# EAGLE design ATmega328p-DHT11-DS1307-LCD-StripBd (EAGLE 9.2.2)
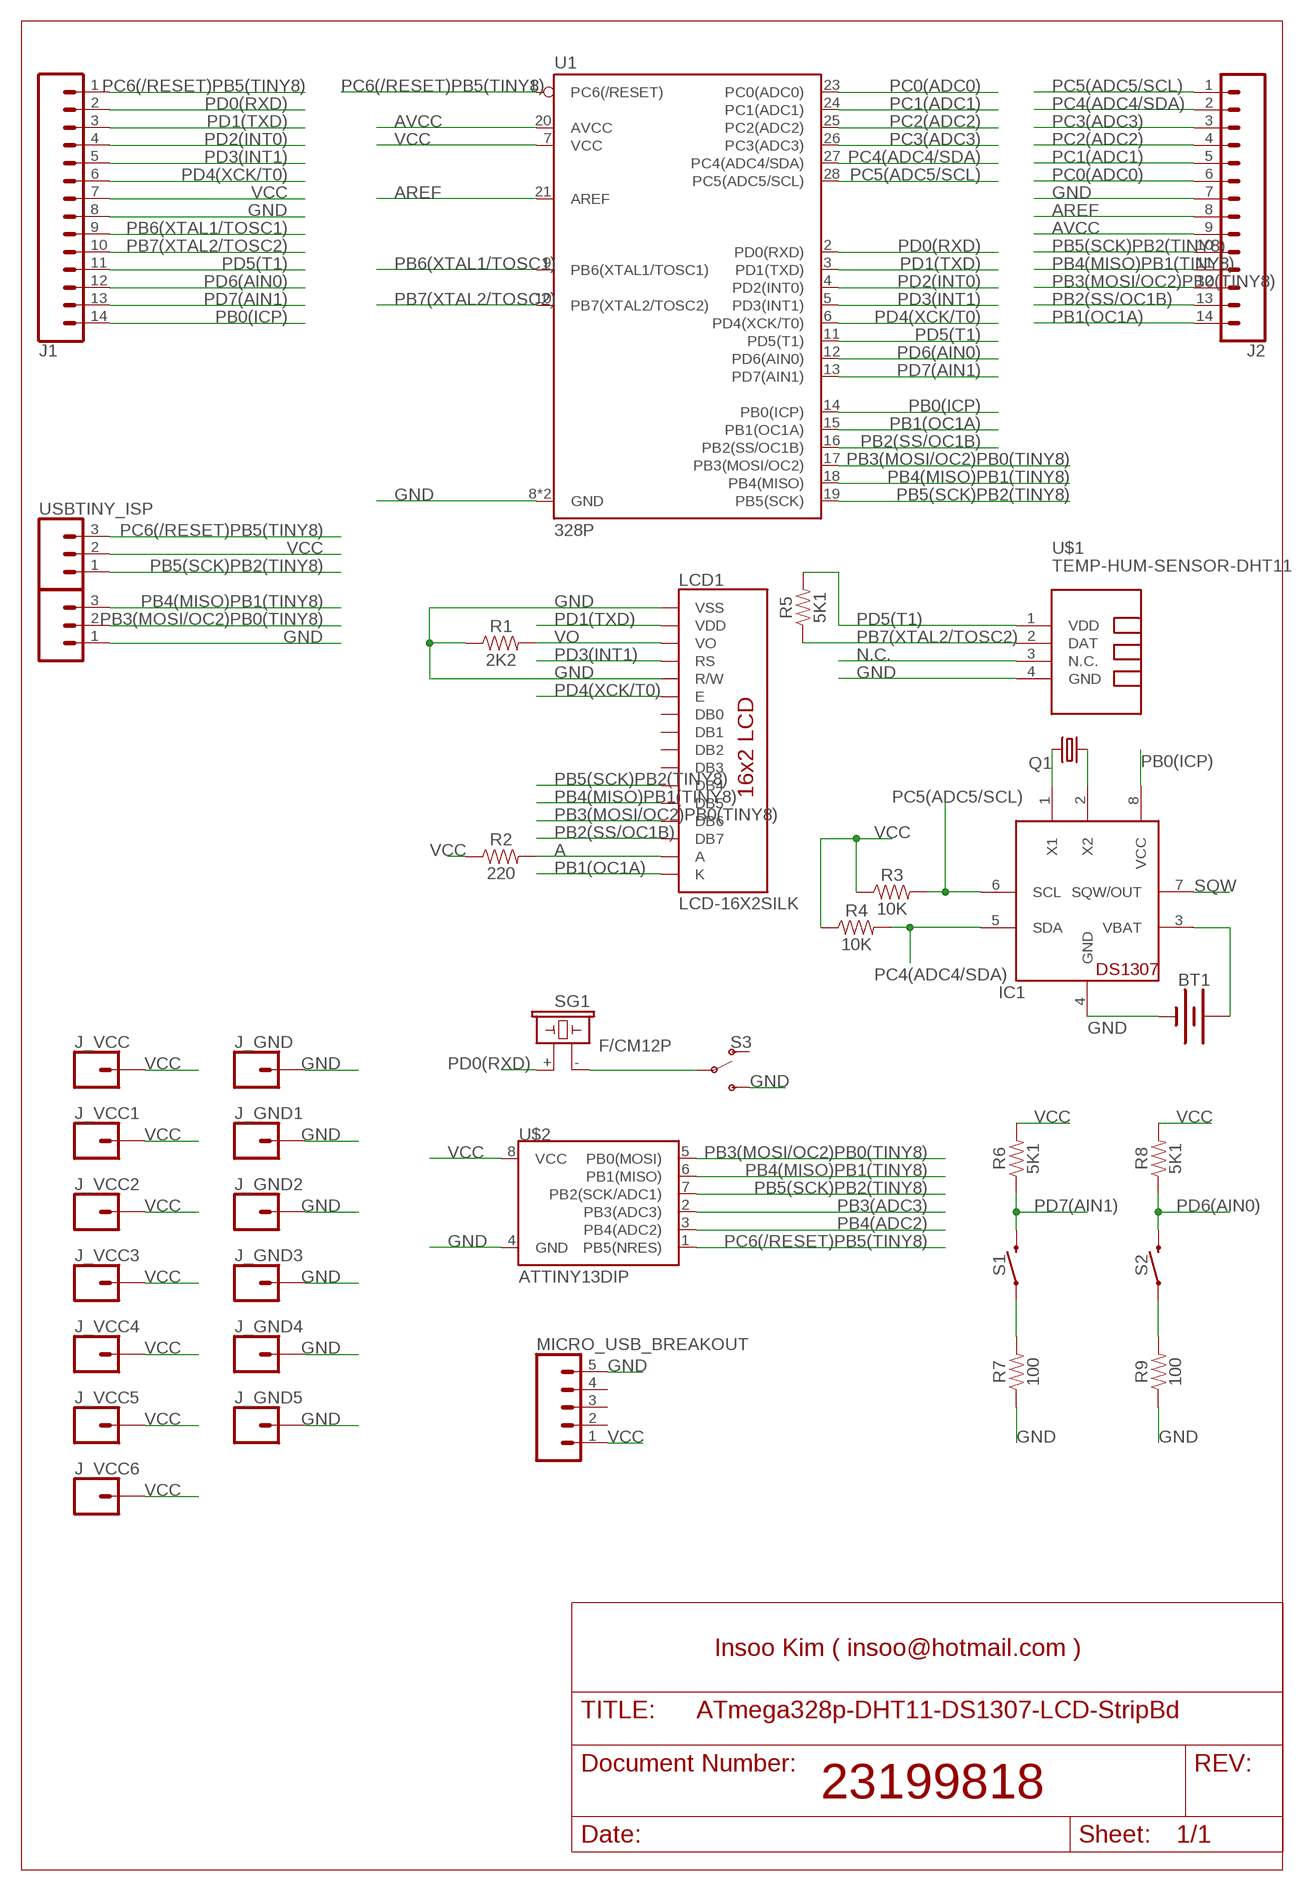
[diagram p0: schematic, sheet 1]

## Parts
BT1  BATTERY-20MM_PTH  [BATTCOM_20MM_PTH]
IC1  DS1307  [DIL08]
J1  CONN_14  [1X14]
J2  CONN_14  [1X14]
J3  455-1750-1-ND  CONN_03  [1X03]
J_GND  CONN_01  [1X01]
J_GND1  CONN_01  [1X01]
J_GND2  CONN_01  [1X01]
J_GND3  CONN_01  [1X01]
J_GND4  CONN_01  [1X01]
J_GND5  CONN_01  [1X01]
J_VCC  CONN_01  [1X01]
J_VCC1  CONN_01  [1X01]
J_VCC2  CONN_01  [1X01]
J_VCC3  CONN_01  [1X01]
J_VCC4  CONN_01  [1X01]
J_VCC5  CONN_01  [1X01]
J_VCC6  CONN_01  [1X01]
LCD1  LCD-16X2SILK  [LCD-16X2]
MICRO_USB_BREAKOUT  CONN_05  [1X05]
Q1  CRYSTALTC26H  [TC26H]
R1  2K2  1KOHM-HORIZ-1/4W-5%  [AXIAL-0.3]
R2  220  1KOHM-HORIZ-1/4W-5%  [AXIAL-0.3]
R3  10K  1KOHM-HORIZ-1/4W-5%  [AXIAL-0.3]
R4  10K  1KOHM-HORIZ-1/4W-5%  [AXIAL-0.3]
R5  5K1  1KOHM-HORIZ-1/4W-5%  [AXIAL-0.3]
R6  5K1  1KOHM-HORIZ-1/4W-5%  [AXIAL-0.3]
R7  100  1KOHM-HORIZ-1/4W-5%  [AXIAL-0.3]
R8  5K1  1KOHM-HORIZ-1/4W-5%  [AXIAL-0.3]
R9  100  1KOHM-HORIZ-1/4W-5%  [AXIAL-0.3]
S1  MOMENTARY-SWITCH-SPST-PTH-12MM  [TACTILE_SWITCH_PTH_12MM]
S2  MOMENTARY-SWITCH-SPST-PTH-12MM  [TACTILE_SWITCH_PTH_12MM]
S3  SWITCH-SPDT-PTH-11.6X4.0MM  [SWITCH_SPDT_PTH_11.6X4.0MM]
SG1  F/CM12P  [F/CM12P]
U1  328P  ATMEGA328P_PDIP  [DIP28]
U$1  TEMP-HUM-SENSOR-DHT11  [TEMP-HUM-SENSOR-DHT11]
U$2  ATTINY13DIP  [DIP08_MCU]
USBTINY_ISP  455-1750-1-ND  CONN_03  [1X03]

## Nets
A: LCD1.15(A) R2.P$2
AREF: J2.8 U1.21(AREF)
AVCC: J2.9 U1.20(AVCC)
GND: BT1.2(-) IC1.4(GND) J1.8 J2.7 J3.1 J_GND1.1 J_GND2.1 J_GND3.1 J_GND4.1 J_GND5.1 J_GND.1 LCD1.1(VSS) LCD1.5(R/W) MICRO_USB_BREAKOUT.5 R1.P$1 R7.P$1 R9.P$1 S3.3(S) U1.8(GND) U1.22(GND) U$1.4(GND) U$2.4(GND)
N$2: S3.2(P) SG1.-
N$40: R7.P$2 S1.1
N$54: IC1.2(X2) Q1.1
N$55: IC1.1(X1) Q1.2
N$56: R9.P$2 S2.1
N$58: BT1.1(+) IC1.3(VBAT)
N.C.: U$1.3(N.C.)
PB0(ICP): IC1.8(VCC) J1.14 U1.14(PB0(ICP))
PB1(OC1A): J2.14 LCD1.16(K) U1.15(PB1(OC1A))
PB2(SS/OC1B): J2.13 LCD1.14(DB7) U1.16(PB2(SS/OC1B))
PB3(ADC3): U$2.2(PB3(ADC3))
PB3(MOSI/OC2)PB0(TINY8): J2.12 J3.2 LCD1.13(DB6) U1.17(PB3(MOSI/OC2)) U$2.5(PB0(MOSI))
PB4(ADC2): U$2.3(PB4(ADC2))
PB4(MISO)PB1(TINY8): J2.11 J3.3 LCD1.12(DB5) U1.18(PB4(MISO)) U$2.6(PB1(MISO))
PB5(SCK)PB2(TINY8): J2.10 LCD1.11(DB4) U1.19(PB5(SCK)) U$2.7(PB2(SCK/ADC1)) USBTINY_ISP.1
PB6(XTAL1/TOSC1): J1.9 U1.9(PB6(XTAL1/TOSC1))
PB7(XTAL2/TOSC2): J1.10 R5.P$1 U1.10(PB7(XTAL2/TOSC2)) U$1.2(DAT)
PC0(ADC0): J2.6 U1.23(PC0(ADC0))
PC1(ADC1): J2.5 U1.24(PC1(ADC1))
PC2(ADC2): J2.4 U1.25(PC2(ADC2))
PC3(ADC3): J2.3 U1.26(PC3(ADC3))
PC4(ADC4/SDA): IC1.5(SDA) J2.2 R4.P$2 U1.27(PC4(ADC4/SDA))
PC5(ADC5/SCL): IC1.6(SCL) J2.1 R3.P$2 U1.28(PC5(ADC5/SCL))
PC6(/RESET)PB5(TINY8): J1.1 U1.1(PC6(/RESET)) U$2.1(PB5(NRES)) USBTINY_ISP.3
PD0(RXD): J1.2 SG1.+ U1.2(PD0(RXD))
PD1(TXD): J1.3 LCD1.2(VDD) U1.3(PD1(TXD))
PD2(INT0): J1.4 U1.4(PD2(INT0))
PD3(INT1): J1.5 LCD1.4(RS) U1.5(PD3(INT1))
PD4(XCK/T0): J1.6 LCD1.6(E) U1.6(PD4(XCK/T0))
PD5(T1): J1.11 R5.P$2 U1.11(PD5(T1)) U$1.1(VDD)
PD6(AIN0): J1.12 R8.P$1 S2.3 U1.12(PD6(AIN0))
PD7(AIN1): J1.13 R6.P$1 S1.3 U1.13(PD7(AIN1))
SQW: IC1.7(SQW/OUT)
VCC: J1.7 J_VCC1.1 J_VCC2.1 J_VCC3.1 J_VCC4.1 J_VCC5.1 J_VCC6.1 J_VCC.1 MICRO_USB_BREAKOUT.1 R2.P$1 R3.P$1 R4.P$1 R6.P$2 R8.P$2 U1.7(VCC) U$2.8(VCC) USBTINY_ISP.2
VO: LCD1.3(VO) R1.P$2
Unconnected: LCD1.7(DB0) LCD1.8(DB1) LCD1.9(DB2) LCD1.10(DB3) MICRO_USB_BREAKOUT.2 MICRO_USB_BREAKOUT.3 MICRO_USB_BREAKOUT.4 S3.1(O)

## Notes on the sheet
- Insoo Kim ( insoo@hotmail.com )
- 23199818

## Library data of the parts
BT1 = SparkFun-Batteries:BATTERY: Battery - Single Cell; PROD_ID: BATT-09031; SF_SKU: PRT-00783
IC1 = adafruit:DS1307: DS1307 Real time clock (RTC) with battery backup ability. Talk to it via i2c
J1 J2 = SparkFun-Connectors:CONN_14: Multi connection point. Often used as Generic Header-pin footprint for 0.1 inch spaced/style header connections On any of the 0.1 inch spaced packages, you can populate with these: Break Away Headers - Straight (PRT-00116) Break Away Male Headers - Right Angle (PRT-00553) Female Headers (PRT-00115)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
J3 USBTINY_ISP = SparkFun-Connectors:CONN_03: Multi connection point. Often used as Generic Header-pin footprint for 0.1 inch spaced/style header connections On any of the 0.1 inch spaced packages, you can populate with these: Break Away Headers - Straight (PRT-00116) Break Away Male Headers - Right Angle (PRT-00553) Female Headers (PRT-00115)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; PROD_ID: XXX-00000
J_GND J_GND1-J_GND5 J_VCC J_VCC1-J_VCC6 = SparkFun-Connectors:CONN_01: Single connection point. Often used as Generic Header-pin footprint for 0.1 inch spaced/style header connections
LCD1 = SparkFun-Displays:LCD-16X2: Standard text-only 16x2 parallel input LCD Basic 16 character by 2 line display. Typically utilizes the extremely common HD44780 parallel interface chipset SparkFun Products: Basic 16x2 Green Basic 8x2 Green; SF_ID: LCD-00255
MICRO_USB_BREAKOUT = SparkFun-Connectors:CONN_05: Multi connection point. Often used as Generic Header-pin footprint for 0.1 inch spaced/style header connections On any of the 0.1 inch spaced packages, you can populate with these: Break Away Headers - Straight (PRT-00116) Break Away Male Headers - Right Angle (PRT-00553) Female Headers (PRT-00115)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
Q1 = adafruit:CRYSTAL: CRYSTAL; OC_FARNELL: unknown; OC_NEWARK: unknown
R1-R9 = SparkFun-Resistors:1KOHM: 1kΩ resistor; PROD_ID: RES-08380; VALUE: 1k
S1 S2 = SparkFun-Switches:MOMENTARY-SWITCH-SPST: Momentary Switch (Pushbutton) - SPST; PROD_ID: SWCH-09185; SF_SKU: COM-09190
S3 = SparkFun-Switches:SWITCH-SPDT: Single Pole, Double Throw (SPDT) Switch Single-pole, double-throw (SPDT) switch. Variant Overview SMD-AYZ0202 Surface Mount DPDT Switch (COM-00597) Used on e.g. LilyPad Arduino USB - ATmega32U4 Board PTH-11.6X4.0MM SPDT Mini Power Switch (COM-00102) Used on e.g. SparkFun Simon Says - Through-Hole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; PROD_ID: SWCH-08261; SF_SKU: COM-00102
SG1 = buzzer:F/CM12P: BUZZER; OC_FARNELL: unknown; OC_NEWARK: unknown
U1 = SparkFun-IC-Microcontroller:ATMEGA328P_PDIP: Atmel 328P Through hole ATMEGA328P uC used in the Arduino 32kb flash, 1k EEPROM, 2k SRAM Datasheet SparkFun Products Storefront component: AVR 28 Pin 20MHz 32K 6A/D - ATMega328P (COM-09061) SparkFun Simon Says - Through-Hole Soldering Kit (KIT-10547) SparkFun Learn to Solder - Simon Says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; PROD_ID: IC-09136
U$1 = diy-modules:TEMP-HUM-SENSOR-DHT11: DHT11 - digital humidity & temperature sensor DHT11 datasheet available here: https://akizukidenshi.com/download/ds/aosong/DHT11.pdf Click here to find device on ebay.com
U$2 = SparkFun-Retired:ATTINY13: ATTINY13 Retired

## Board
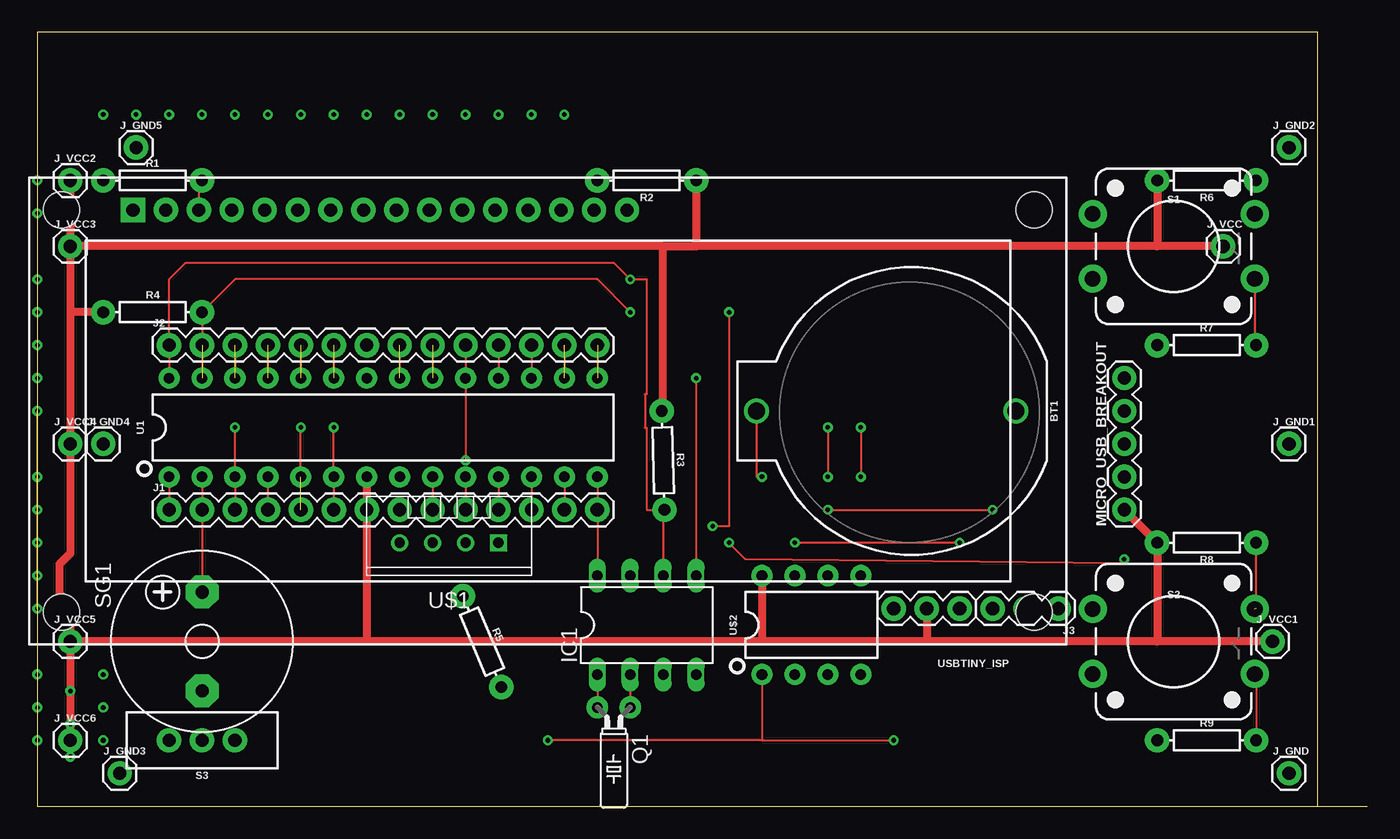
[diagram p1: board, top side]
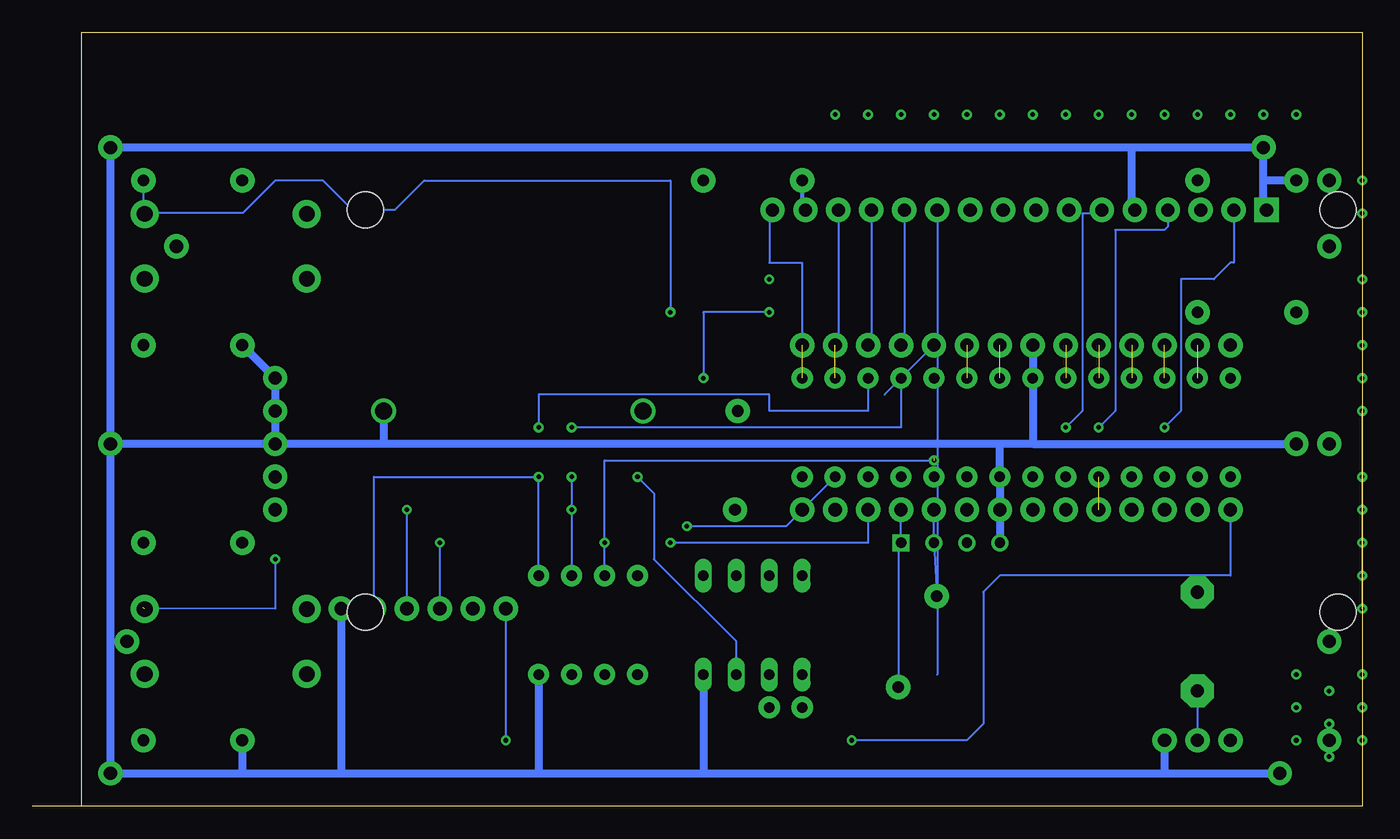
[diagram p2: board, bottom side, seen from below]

Size 102.54 x 59.68 mm. Coordinates in mm from the lower left corner, seen from the top.
Outline: 98.73,0 98.73,59.68 0,59.68 0,0 98.73,0
Outline: 98.73,0 102.54,0
Outline: 3.81,0 101.27,0
Copper layers (1*16): Top 0.035mm / dielectric 1.5mm / Bottom 0.035mm
Design rules "default": minimum track width 6mil, minimum drill 0.35mm, track to track 6mil, track to pad 6mil, pad to pad 6mil, via to via 6mil, smd to smd 6mil, copper to edge 40mil, drill to drill 6mil, minimum pad ring 10mil, minimum via ring 8mil, stop-mask expansion 4mil, vias tented up to drill 0mil, thermal gap 10mil

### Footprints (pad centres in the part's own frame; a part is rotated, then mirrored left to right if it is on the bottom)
BATTCOM_20MM_PTH = drill 1.3: 1 11.85,0; 2 -8.15,0
DIL08 = drill 0.813 long: 1 -3.81,-3.81; 2 -1.27,-3.81; 3 1.27,-3.81; 4 3.81,-3.81; 5 3.81,3.81; 6 1.27,3.81; 7 -1.27,3.81; 8 -3.81,3.81
1X14 = drill 1.016 pad 1.88: 1 0,0; 2 2.54,0; 3 5.08,0; 4 7.62,0; 5 10.16,0; 6 12.7,0; 7 15.24,0; 8 17.78,0; 9 20.32,0; 10 22.86,0; 11 25.4,0; 12 27.94,0; 13 30.48,0; 14 33.02,0
1X03 = drill 1.016 pad 1.88: 1 0,0; 2 2.54,0; 3 5.08,0
1X01 = drill 1.016 pad 1.88: 1 0,0
LCD-16X2 = drill 1.016 pad 1.88 square: 1 -32,15.5 | drill 1.016 pad 1.88: 2 -29.46,15.5; 3 -26.92,15.5; 4 -24.38,15.5; 5 -21.84,15.5; 6 -19.3,15.5; 7 -16.76,15.5; 8 -14.22,15.5; 9 -11.68,15.5; 10 -9.14,15.5; 11 -6.6,15.5; 12 -4.06,15.5; 13 -1.52,15.5; 14 1.02,15.5; 15 3.56,15.5; 16 6.1,15.5 | hole 2.8: -37.5,15.5; -37.5,-15.5; 37.5,15.5; 37.5,-15.5
1X05 = drill 1.016 pad 1.88: 1 0,0; 2 2.54,0; 3 5.08,0; 4 7.62,0; 5 10.16,0
TC26H = drill 0.813 pad 1.676: 1 -1.27,0; 2 1.27,0
AXIAL-0.3 = drill 0.9 pad 1.88: P$1 -3.81,0; P$2 3.81,0
TACTILE_SWITCH_PTH_12MM = drill 1.2 pad 2.159: 1 6.25,-2.5; 2 -6.25,-2.5; 3 6.25,2.5; 4 -6.25,2.5
SWITCH_SPDT_PTH_11.6X4.0MM = drill 1.016 pad 1.88: 1 0,2.54; 2 0,0; 3 0,-2.54
F/CM12P = drill 1.016 pad 2.54 octagon: + 3.81,0; - -3.81,0
DIP28 = drill 0.813 pad 1.626: 1 -16.51,-3.81; 2 -13.97,-3.81; 3 -11.43,-3.81; 4 -8.89,-3.81; 5 -6.35,-3.81; 6 -3.81,-3.81; 7 -1.27,-3.81; 8 1.27,-3.81; 9 3.81,-3.81; 10 6.35,-3.81; 11 8.89,-3.81; 12 11.43,-3.81; 13 13.97,-3.81; 14 16.51,-3.81; 15 16.51,3.81; 16 13.97,3.81; 17 11.43,3.81; 18 8.89,3.81; 19 6.35,3.81; 20 3.81,3.81; 21 1.27,3.81; 22 -1.27,3.81; 23 -3.81,3.81; 24 -6.35,3.81; 25 -8.89,3.81; 26 -11.43,3.81; 27 -13.97,3.81; 28 -16.51,3.81
TEMP-HUM-SENSOR-DHT11 = drill 0.8 square: 1 -3.81,0 | drill 0.8: 2 -1.27,0; 3 1.27,0; 4 3.81,0
DIP08_MCU = drill 0.813 pad 1.626: 1 -3.81,-3.81; 2 -1.27,-3.81; 3 1.27,-3.81; 4 3.81,-3.81; 5 3.81,3.81; 6 1.27,3.81; 7 -1.27,3.81; 8 -3.81,3.81

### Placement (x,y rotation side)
BT1  67.31,30.48 180 top
IC1  46.99,13.97 0 top
J1  10.16,22.86 0 top
J2  10.16,35.56 0 top
J3  78.74,15.24 180 top
J_GND  96.52,2.54 0 top
J_GND1  96.52,27.94 0 top
J_GND2  96.52,50.8 0 top
J_GND3  6.35,2.54 0 top
J_GND4  5.08,27.94 0 top
J_GND5  7.62,50.8 0 top
J_VCC  91.44,43.18 0 top
J_VCC1  95.25,12.7 0 top
J_VCC2  2.54,48.26 0 top
J_VCC3  2.54,43.18 0 top
J_VCC4  2.54,27.94 0 top
J_VCC5  2.54,12.7 0 top
J_VCC6  2.54,5.08 0 top
LCD1  39.37,30.48 0 top
MICRO_USB_BREAKOUT  83.82,22.86 90 top
Q1  44.45,7.62 180 top
R1  8.89,48.26 0 top
R2  46.99,48.26 180 top
R3  48.26,26.67 271.6 top
R4  8.89,38.1 0 top
R5  34.29,12.7 292.9 top
R6  90.17,48.26 180 top
R7  90.17,35.56 0 top
R8  90.17,20.32 180 top
R9  90.17,5.08 0 top
S1  87.63,43.18 0 top
S2  87.63,12.7 0 top
S3  12.7,5.08 90 top
SG1  12.7,12.7 90 top
U1  26.67,29.21 0 top
U$1  31.75,20.32 180 top
U$2  59.69,13.97 0 top
USBTINY_ISP  71.12,15.24 180 top

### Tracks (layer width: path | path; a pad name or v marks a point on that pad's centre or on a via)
A
  Bottom 0.305: R2.P$2 43.18,46.23 LCD1.15
AREF  (2 unrouted)
  Top 0.152: J2.8 U1.21
AVCC  (2 unrouted)
  Top 0.152: J2.9 U1.20
GND
  Bottom 0.61: J_GND1.1 J_GND.1 86.36,2.54 | J_GND1.1 J_GND2.1 17.78,50.8 | 50.8,2.54 15.24,2.54 | 15.24,2.54 J_GND3.1 | 86.36,2.54 78.74,2.54 | 78.74,2.54 63.5,2.54 | 63.5,2.54 50.8,2.54 | 17.78,50.8 J_GND5.1 7.62,48.26 | 25.4,27.94 J_GND4.1 | 25.4,27.94 27.94,27.94 | 27.94,27.94 75.46,27.94 | 75.46,27.94 83.82,27.94 | 83.82,27.94 J_GND1.1 | LCD1.1 7.62,45.98 7.62,48.26 | LCD1.5 17.78,45.98 17.78,50.8 | 27.94,27.94 U1.8 J1.8 U$1.4 | J2.7 U1.22 25.4,27.94 | BT1.2 75.46,27.94 | IC1.4 50.8,2.54 | R7.P$1 MICRO_USB_BREAKOUT.5 83.82,27.94 | R9.P$1 86.36,2.54 | U$2.4 63.5,2.54 | R1.P$1 7.62,48.26 | S3.3 15.24,2.54 | J3.1 78.74,2.54
N$1  (via drill 0.35)
  other vias: 0,10.16
N$2
  Bottom 0.152: SG1.- S3.2
N$5  (via drill 0.35)
  other vias: 12.7,53.34
N$6  (via drill 0.35)
  other vias: 10.16,53.34
N$7  (via drill 0.35)
  other vias: 7.62,53.34
N$8  (via drill 0.35)
  other vias: 5.08,53.34
N$9  (via drill 0.35)
  other vias: 0,5.08
N$10  (via drill 0.35)
  other vias: 15.24,53.34
N$11  (via drill 0.35)
  other vias: 0,33.02
N$12  (via drill 0.35)
  other vias: 0,35.56
N$13  (via drill 0.35)  (1 unrouted)
  other vias: 0,15.24 0,30.48
N$14  (via drill 0.35)
  other vias: 0,17.78
N$15  (via drill 0.35)
  other vias: 0,20.32
N$16  (via drill 0.35)
  other vias: 0,22.86
N$17  (via drill 0.35)
  other vias: 0,25.4
N$18  (via drill 0.35)
  other vias: 0,38.1
N$19  (via drill 0.35)
  other vias: 0,40.64
N$20  (via drill 0.35)
  other vias: 0,45.72
N$21  (via drill 0.35)
  other vias: 0,48.26
N$22  (via drill 0.35)
  other vias: 0,7.62
N$23  (via drill 0.35)
  other vias: 17.78,53.34
N$24  (via drill 0.35)
  other vias: 20.32,53.34
N$25  (via drill 0.35)
  other vias: 22.86,53.34
N$26  (via drill 0.35)
  other vias: 25.4,53.34
N$27  (via drill 0.35)
  other vias: 27.94,53.34
N$28  (via drill 0.35)
  other vias: 30.48,53.34
N$29  (via drill 0.35)
  other vias: 33.02,53.34
N$30  (via drill 0.35)
  other vias: 35.56,53.34
N$31  (via drill 0.35)
  other vias: 38.1,53.34
N$32  (via drill 0.35)
  other vias: 40.64,53.34
N$40
  Top 0.152: S1.1 93.88,35.66 R7.P$2
N$45  (via drill 0.35)
  other vias: 2.54,3.81
N$46  (via drill 0.35)
  other vias: 2.54,6.35
N$47  (via drill 0.35)
  other vias: 2.54,8.89
N$48  (via drill 0.35)
  other vias: 5.08,10.16
N$49  (via drill 0.35)
  other vias: 5.08,7.62
N$50  (via drill 0.35)
  other vias: 5.08,5.08
N$54
  Top 0.152: IC1.2 Q1.1
N$55
  Top 0.152: IC1.1 Q1.2
N$56
  Top 0.152: R9.P$2 93.98,10.1 S2.1
N$58  (via drill 0.35)
  Top 0.152: BT1.1 55.46,25.4 v55.88,25.4
  Bottom 0.152: IC1.3 48.26,12.7 54.61,19.05 54.61,24.13 v55.88,25.4
PB0(ICP)
  Top 0.152: U1.14 J1.14 IC1.8
PB1(OC1A)  (2 unrouted)
  Top 0.152: J2.14 U1.15
  Bottom 0.152: LCD1.16 45.72,45.73 45.72,41.91 43.18,41.91 J2.14
PB2(SS/OC1B)  (2 unrouted)
  Top 0.152: J2.13 U1.16
  Bottom 0.152: LCD1.14 40.39,35.81 J2.13
  Bottom 0.305: U1.16 40.39,33.27
PB3(MOSI/OC2)PB0(TINY8)  (via drill 0.35)
  Top 0.152: J2.12 U1.17 | v63.5,29.21 v63.5,25.4
  Bottom 0.152: LCD1.13 37.85,35.81 J2.12 | U1.17 38.1,30.48 45.72,30.48 45.72,31.75 63.5,31.75 v63.5,29.21 | U$2.5 v63.5,25.4 76.2,25.4 J3.2
  Bottom 0.305: U1.17 37.85,33.27
PB4(MISO)PB1(TINY8)  (via drill 0.35)
  Top 0.152: J2.11 U1.18 | v60.96,29.21 v60.96,25.4 | v60.96,22.86 v73.66,22.86
  Bottom 0.152: LCD1.12 35.31,35.81 J2.11 | U1.18 35.56,29.21 v60.96,29.21 | v60.96,25.4 v60.96,22.86 U$2.6 | J3.3 v73.66,22.86
  Bottom 0.305: U1.18 35.31,33.27
PB5(SCK)PB2(TINY8)  (via drill 0.35)  (1 unrouted)
  Top 0.152: J2.10 U1.19 33.02,26.87 | v71.12,20.32 v58.42,20.32
  Bottom 0.152: LCD1.11 32.77,35.81 | 32.77,35.81 32.77,10.16 | 32.77,35.81 J2.10 36.83,31.75 | v33.02,26.67 58.42,26.67 v58.42,20.32 U$2.7 | USBTINY_ISP.1 v71.12,20.32
  Bottom 0.305: U1.19 32.77,33.27
PB6(XTAL1/TOSC1)
  Top 0.152: U1.9 J1.9
PB7(XTAL2/TOSC2)
  Top 0.152: U1.10 J1.10
  Bottom 0.152: J1.10 U$1.2 R5.P$1
PC0(ADC0)  (2 unrouted)
  Top 0.152: J2.6 U1.23
PC1(ADC1)  (2 unrouted)
  Top 0.152: J2.5 U1.24
PC2(ADC2)  (2 unrouted)
  Top 0.152: J2.4 U1.25
PC3(ADC3)  (2 unrouted)
  Top 0.152: J2.3 U1.26
PC4(ADC4/SDA)  (via drill 0.35)  (1 unrouted)
  Top 0.152: U1.27 J2.2 R4.P$2 15.24,40.64 43.18,40.64 v45.72,38.1 | v50.8,33.02 IC1.5
  Bottom 0.152: v45.72,38.1 50.8,38.1 v50.8,33.02
PC5(ADC5/SCL)  (via drill 0.35)
  Top 0.152: U1.28 J2.1 10.16,40.64 11.43,41.91 44.45,41.91 v45.72,40.64 46.99,40.64 46.99,31.78 46.85,31.78 46.85,29.18 46.99,29.18 46.99,22.86 48.26,22.86 | R3.P$2 48.26,22.86 | 48.26,22.86 IC1.6
  Bottom 0.152: 48.1,17.94 IC1.6
PC6(/RESET)PB5(TINY8)  (via drill 0.35)
  Top 0.152: U1.1 J1.1 | U$2.1 55.88,5.08 | 55.88,5.08 v39.37,5.08 | 55.88,5.08 v66.04,5.08
  Bottom 0.152: J1.1 10.16,17.78 27.94,17.78 29.21,16.51 29.21,6.35 30.48,5.08 v39.37,5.08 | USBTINY_ISP.3 v66.04,5.08
PD0(RXD)
  Top 0.152: U1.2 J1.2 SG1.+
PD1(TXD)  (via drill 0.35)
  Top 0.152: v15.24,29.21 U1.3 J1.3
  Bottom 0.152: 10.16,45.73 LCD1.2 9.91,41.91 10.16,41.91 11.43,40.64 13.97,40.64 13.97,30.48 v15.24,29.21
PD2(INT0)
  Top 0.152: U1.4 J1.4
PD3(INT1)  (via drill 0.35)  (1 unrouted)
  Top 0.152: U1.5 v20.32,29.21
  Bottom 0.152: 15.24,45.73 LCD1.4 14.99,44.7 15.24,44.45 19.05,44.45 19.05,30.48 v20.32,29.21
PD4(XCK/T0)  (via drill 0.35)
  Top 0.152: J1.6 U1.6 v22.86,29.21
  Bottom 0.152: LCD1.6 20.07,45.72 21.59,45.72 21.59,30.48 v22.86,29.21
PD5(T1)
  Top 0.152: U1.11 J1.11 35.77,22.86
  Bottom 0.152: R5.P$2 35.77,20.11 U$1.1 J1.11
PD6(AIN0)  (via drill 0.35)  (1 unrouted)
  Top 0.152: U1.12 J1.12 | 93.98,15.3 R8.P$1 | v53.34,20.32 54.61,19.05 83.5,18.73 v83.82,19.05
  Bottom 0.152: J1.12 38.1,20.32 v53.34,20.32 | v83.82,19.05 83.82,15.24 S2.3
PD7(AIN1)  (via drill 0.35)
  Top 0.152: U1.13 J1.13 | v53.34,38.1 53.34,21.59 v52.07,21.59
  Bottom 0.152: U1.13 44.45,21.59 v52.07,21.59 | v53.34,38.1 53.34,48.26 72.33,48.26 74.57,46.03 77.9,46.03 80.14,48.26 83.82,48.26 86.33,45.75 93.95,45.75 | R6.P$1 93.98,45.78 93.95,45.75 | S1.3 93.95,45.75
VCC
  Top 0.61: J_VCC5.1 J_VCC6.1 | 48.26,43.18 J_VCC3.1 | 48.26,43.18 50.8,43.18 | J_VCC.1 86.36,43.18 | 86.36,43.18 50.8,43.18 | 25.4,12.7 J_VCC5.1 | J_VCC1.1 86.36,12.7 | 86.36,12.7 68.58,12.7 | 68.58,12.7 55.88,12.7 | 55.88,12.7 25.4,12.7 | J_VCC3.1 2.54,38.1 | 2.54,38.1 J_VCC4.1 2.54,19.5 1.69,18.65 1.69,16.39 2.54,15.54 J_VCC5.1 | R2.P$1 50.8,43.18 | U1.7 J1.7 25.4,12.7 | R4.P$1 2.54,38.1 | R3.P$1 48.26,30.48 48.26,43.18 | J_VCC2.1 J_VCC3.1 | R6.P$2 86.36,43.18 | 86.36,12.7 R8.P$2 MICRO_USB_BREAKOUT.1 | U$2.8 55.88,12.7 | USBTINY_ISP.2 68.58,12.7
VO
  Top 0.152: R1.P$2 12.45,48.01 LCD1.3

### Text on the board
tValues: 1 2 3 4 5 | 6 7 8 9 10 | 1 2 3 4 5 | 6 7 8 9 20 | 1 2 3 4 5 | 6 7 8 9 30 | 1 2 3 4 35 | 36 | 1 2 | 1 2 3 4 5 | 1 2 3 4 5 | 1 2 3 4 5 | 1 2 3 | 1 2 3 4 5 | 6 7 8 9 10 | 1 2 3 4 5 | 6 7 8 9 20 | 1 2 3 4 5 | 6 7 8 9 30 | 1 2 3 4 35 | 36

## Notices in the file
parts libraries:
SparkFun-IC-Microcontroller: Licensing: Creative Commons ShareAlike 4.0 International - https://creativecommons.org/licenses/by-sa/4.0
diy-modules: Released under the Creative Commons Attribution 4.0 International License: http://creativecommons.org/licenses/by/4.0
